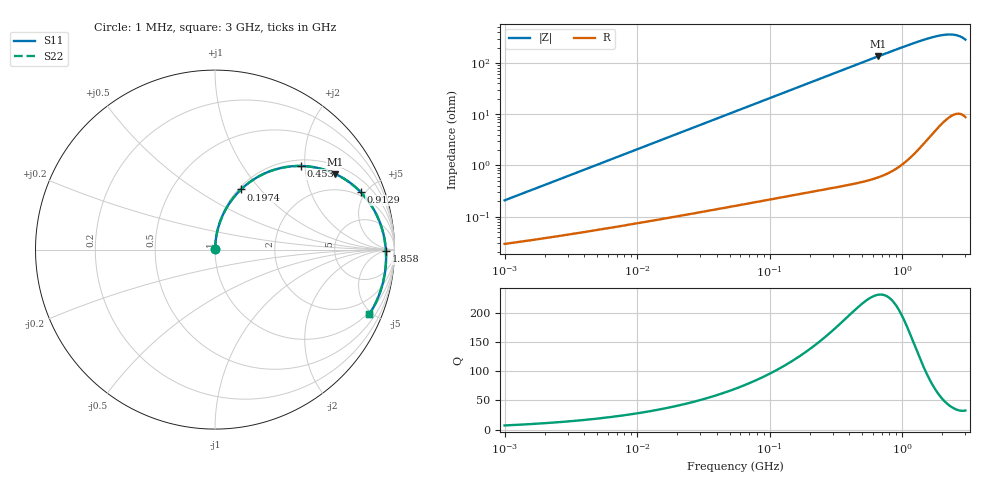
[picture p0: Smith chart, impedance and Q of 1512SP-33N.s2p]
# MHz  S  MA  R  50
!Freq  MagS11  AngS11  MagS21  AngS21  MagS12  AngS12  MagS22  AngS22
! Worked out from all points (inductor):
!   801 points, 1 MHz to 3 GHz, reference 50 ohm
!   read as one part in series: L = 32.8 nH near 1.041 MHz
!   highest Q = 231 at 656.1 MHz (marker M1), where L = 32.6 nH
!   S11 on the Smith chart (normalised r, x): 1 MHz: 1.00, +0.00; 197.4 MHz: 1.03, +0.79; 453 MHz: 1.13, +1.90; 912.9 MHz: 1.72, +4.62; 1.858 GHz: 40, -7; 3 GHz: 0.88, -4.82
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1  0.002013 81.5  0.9997 -0.1  0.9997 -0.1  0.002013 81.5
3.824029  0.007631 85.8  0.9995 -0.5  0.9995 -0.5  0.007631 85.8
14.47755  0.02882 86.5  0.9987 -1.8  0.9987 -1.8  0.02882 86.5
30.06344  0.05974 85.2  0.997 -3.7  0.997 -3.7  0.05973 85.2
54.81117  0.1084 82.5  0.9925 -6.7  0.9925 -6.7  0.1084 82.5
114.9635  0.2228 75.7  0.9726 -13.8  0.9726 -13.8  0.2228 75.7
153.6837  0.2921 71.3  0.9539 -18.2  0.9539 -18.2  0.292 71.3
197.3818  0.365 66.6  0.9283 -22.9  0.9283 -22.9  0.3649 66.6
209.5995  0.3843 65.3  0.9204 -24.2  0.9204 -24.2  0.3842 65.3
300.5304  0.5122 56.5  0.8558 -33.2  0.8558 -33.2  0.5119 56.5
374.5642  0.5962 50.2  0.7997 -39.5  0.7997 -39.5  0.5959 50.2
453.0254  0.6678 44.3  0.7412 -45.5  0.7412 -45.5  0.6674 44.3
542.4649  0.7315 38.5  0.6787 -51.3  0.6787 -51.3  0.731 38.5
656.0968  0.7913 32.2  0.6082 -57.5  0.6082 -57.5  0.7908 32.2
793.5315  0.8417 26.1  0.5366 -63.7  0.5366 -63.7  0.8411 26.1
912.9029  0.8723 21.6  0.4852 -68.1  0.4852 -68.1  0.8716 21.6
1308.949  0.9272 10.5  0.368 -79.0  0.368 -79.0  0.9264 10.5
1858.12  0.9526 -0.5  0.2885 -89.6  0.2885 -89.6  0.9519 -0.5
2159.143  0.9558 -5.8  0.2713 -94.5  0.2713 -94.5  0.9552 -5.8
2434.712  0.9541 -10.8  0.27 -99.1  0.27 -99.1  0.9537 -10.8
2691.034  0.9481 -15.7  0.2828 -103.8  0.2828 -103.8  0.948 -15.7
3000  0.9322 -22.7  0.322 -110.7  0.322 -110.7  0.9327 -22.7
